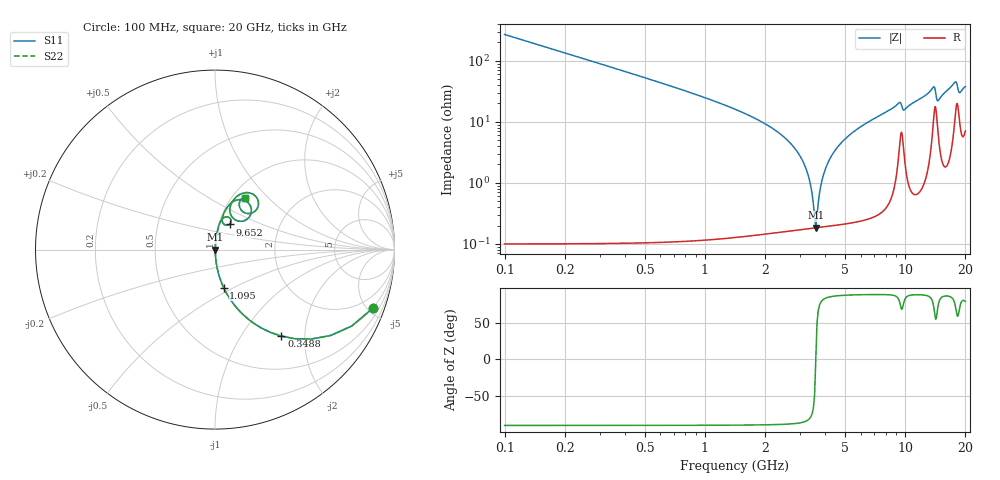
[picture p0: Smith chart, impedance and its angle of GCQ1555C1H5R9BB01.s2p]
!Murata Part Number: GCQ1555C1H5R9BB01
!These Parameters are Measured in Series Mode Connection
!Data Generated on Jan 08, 2026
!  o--ll--o
!Port1  Port2
!  o------o
!Operation Temp=25[degC], DC Bias Voltage=0[V]
!Freq. Start=100[MHz] Stop=20[GHz] 401[Steps]
# Hz S RI R 50
!Freq.(Hz) S11(Real) S11(Imag) S21(Real) S21(Imag) S12(Real) S12(Imag) S22(Real) S22(Imag)
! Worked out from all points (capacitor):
!   401 points, 100 MHz to 20 GHz, reference 50 ohm
!   read as one part in series: C = 5.9 pF near 199.5 MHz
!   lowest |Z| = 183 mohm at 3.583 GHz (marker M1)
!   series resonance near 3.58 GHz, so ESL is about 340 pH
!   S11 on the Smith chart (normalised r, x): 100 MHz: 1.00, -5.39; 348.8 MHz: 1.00, -1.53; 1.095 GHz: 1.00, -0.45; 9.652 GHz: 1.13, +0.32; 20 GHz: 1.14, +0.74
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1e8  0.8789 -0.326  0.1211 0.326  0.1211 0.326  0.8789 -0.326
3.4875e8  0.37 -0.4821  0.63 0.4821  0.63 0.4821  0.37 -0.4821
6.4725e8  0.1404 -0.3461  0.8596 0.3461  0.8596 0.3461  0.1404 -0.3461
1.095e9  0.0485 -0.2121  0.9515 0.2121  0.9515 0.2121  0.0485 -0.2121
2.83625e9  0.00291 -0.0353  0.9971 0.0353  0.9971 0.0353  0.00291 -0.0353
3.23425e9  0.00199 -0.0153  0.998 0.0153  0.998 0.0153  0.00199 -0.0153
3.43325e9  0.00184 -0.00629  0.9982 0.00629  0.9982 0.00629  0.00184 -0.00629
3.5825e9  0.00183 0.000121  0.9982 -0.000121  0.9982 -0.000121  0.00183 0.000121
3.93075e9  0.0021 0.0141  0.9979 -0.0141  0.9979 -0.0141  0.0021 0.0141
4.42825e9  0.00305 0.0324  0.997 -0.0324  0.997 -0.0324  0.00305 0.0324
5.32375e9  0.00601 0.0617  0.994 -0.0617  0.994 -0.0617  0.00601 0.0617
6.7665e9  0.0136 0.104  0.9864 -0.104  0.9864 -0.104  0.0136 0.104
9.30375e9  0.0648 0.1827  0.9352 -0.1827  0.9352 -0.1827  0.0648 0.1827
9.652e9  0.081 0.1402  0.919 -0.1402  0.919 -0.1402  0.081 0.1402
1.005e10  0.042 0.1533  0.958 -0.1533  0.958 -0.1533  0.042 0.1533
1.338325e10  0.1151 0.2743  0.8849 -0.2743  0.8849 -0.2743  0.1151 0.2743
1.39305e10  0.192 0.252  0.808 -0.252  0.808 -0.252  0.192 0.252
1.45275e10  0.1063 0.1704  0.8937 -0.1704  0.8937 -0.1704  0.1063 0.1704
1.67165e10  0.1301 0.3021  0.8699 -0.3021  0.8699 -0.3021  0.1301 0.3021
1.7811e10  0.2272 0.2961  0.7728 -0.2961  0.7728 -0.2961  0.2272 0.2961
1.865675e10  0.1524 0.2136  0.8476 -0.2136  0.8476 -0.2136  0.1524 0.2136
2e10  0.1658 0.2886  0.8342 -0.2886  0.8342 -0.2886  0.1658 0.2886
